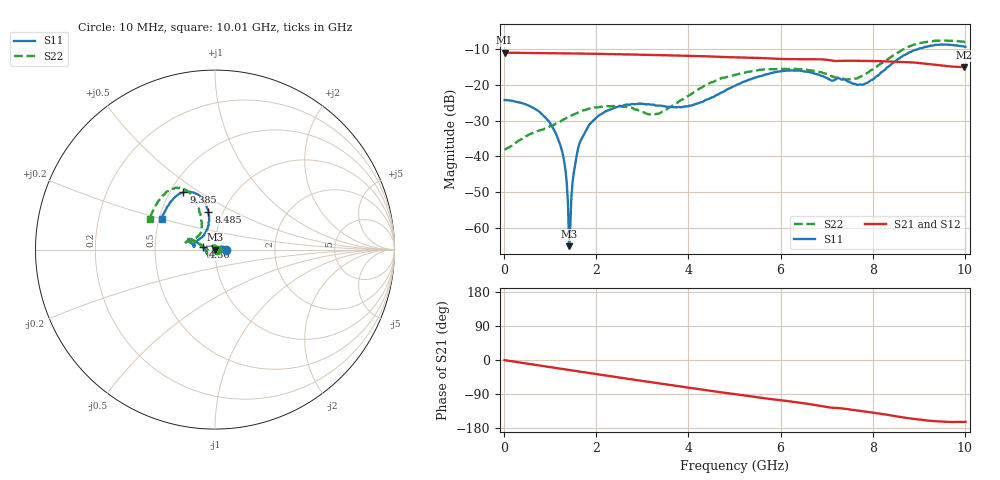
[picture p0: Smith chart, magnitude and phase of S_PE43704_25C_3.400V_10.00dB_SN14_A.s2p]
! Device ID: PE43704
! Dir: z:\PE43704\PE43704_Char_1_20130516\PE43704\AMB\3p400V\10p00dB
! Serial: 14
! Insertion: A
! Impedance: 50 ohm
! Temp: Amb
! VDD: 3.400V
! Attenuation Step: 10.00dB
! IDD: 1.141097e-01mA
#  Hz  S  RI  R  50
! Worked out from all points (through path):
!   401 points, 10 MHz to 10.01 GHz, reference 50 ohm
!   highest |S21| = -10.96 dB at 10 MHz (marker M1); lowest = -15.0 dB at 9.985 GHz (marker M2)
!   group delay of S21, straight-line fit = 47.1 ps
!   lowest |S11| = -65.2 dB at 1.41 GHz (marker M3), VSWR 1.00, Z = 50 + j0.0419 ohm
!   |S11| at or under -10 dB: start of sweep to 8.97 GHz
!   |S22| runs from -38.2 to -7.5 dB; largest |S21 - S12| = 0.0018
!   S11 on the Smith chart (normalised r, x): 10 MHz: 1.13, +0.00; 4.56 GHz: 0.87, +0.02; 8.485 GHz: 0.85, +0.38; 9.385 GHz: 0.58, +0.43; 10.01 GHz: 0.52, +0.20
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1e7  0.0613 0.00018  0.2831 -0.00107  0.2832 -0.00106  0.0123 0.000382
6.6e8  0.0436 0.0166  0.2737 -0.0609  0.2736 -0.0608  -0.000488 0.0217
1.035e9  0.0226 0.0136  0.2629 -0.0929  0.2628 -0.0928  -0.0179 0.0202
1.285e9  0.00783 0.00588  0.2531 -0.1134  0.2531 -0.1133  -0.03 0.0131
1.385e9  0.00146 0.00165  0.2488 -0.1212  0.2488 -0.1212  -0.034 0.00955
1.41e9  0.000355 0.000419  0.2477 -0.1231  0.2478 -0.1231  -0.035 0.00845
1.46e9  -0.00218 -0.00164  0.2455 -0.1269  0.2455 -0.1268  -0.0367 0.00634
1.51e9  -0.0046 -0.0035  0.2431 -0.1307  0.2432 -0.1306  -0.0383 0.00429
1.56e9  -0.00752 -0.00503  0.2409 -0.1344  0.2409 -0.1344  -0.0399 0.00202
1.685e9  -0.0134 -0.0117  0.2346 -0.1438  0.2346 -0.1436  -0.0434 -0.00333
2.235e9  -0.0284 -0.0331  0.2032 -0.1797  0.2033 -0.1796  -0.0464 -0.0201
3.36e9  -0.0364 -0.0363  0.1245 -0.2303  0.1248 -0.2303  -0.0394 -0.00492
4.56e9  -0.0676 0.013  0.0314 -0.2476  0.032 -0.2475  -0.1028 0.0445
5.01e9  -0.0912 0.0339  -0.000744 -0.2438  -0.000392 -0.2439  -0.1309 0.0445
5.96e9  -0.142 0.0599  -0.0623 -0.2237  -0.0616 -0.2239  -0.1606 0.0451
6.685e9  -0.1423 0.0414  -0.1062 -0.2033  -0.1062 -0.2032  -0.1513 0.0486
7.735e9  -0.0688 0.0745  -0.1523 -0.1554  -0.152 -0.1556  -0.0763 0.1066
8.36e9  -0.0332 0.182  -0.1757 -0.1204  -0.1751 -0.1209  -0.0883 0.2205
8.485e9  -0.0362 0.2101  -0.1796 -0.1112  -0.1788 -0.1122  -0.0989 0.2499
9.385e9  -0.1763 0.3192  -0.1806 -0.0599  -0.1814 -0.0593  -0.2532 0.3302
9.985e9  -0.2918 0.1824  -0.1705 -0.0506  -0.171 -0.0507  -0.3581 0.1798
1.001e10  -0.2964 0.1727  -0.171 -0.0515  -0.1723 -0.0514  -0.362 0.1717
